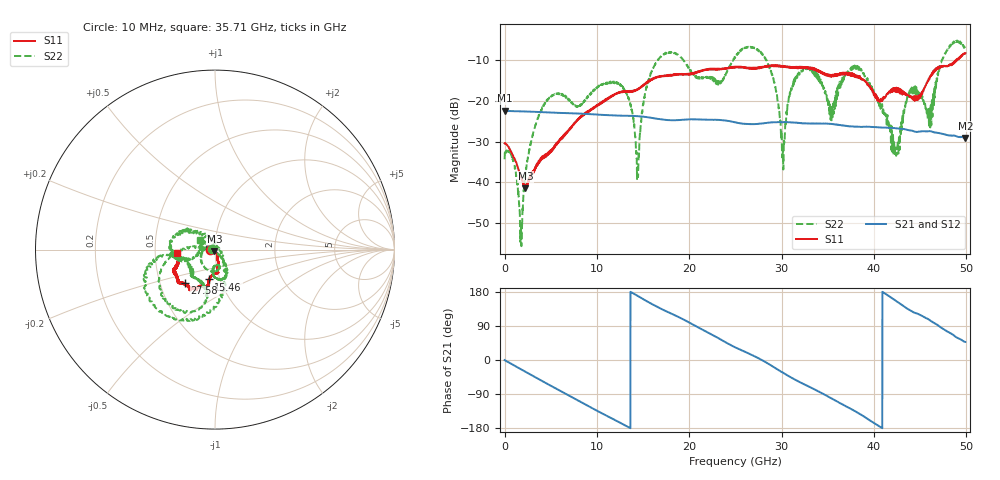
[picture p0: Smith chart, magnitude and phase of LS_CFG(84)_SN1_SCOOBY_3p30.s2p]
!Keysight Technologies,N5245B,MY58422026,A.13.80.08
!Date: Thursday, March 19, 2020 23:53:24
!Correction: S11(Full 2 Port(1,2))
!S21(Full 2 Port(1,2))
!S12(Full 2 Port(1,2))
!S22(Full 2 Port(1,2))
!S2P File: Measurements: S11, S21, S12, S22:
# Hz S DB R 50.0
!freq dBS11 angS11 dBS21 angS21 dBS12 angS12 dBS22 angS22
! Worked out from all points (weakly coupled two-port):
!   4991 points, 10 MHz to 49.91 GHz, reference 50 ohm
!   highest |S21| = -22.43 dB at 10 MHz (marker M1); lowest = -29.1 dB at 49.91 GHz (marker M2)
!   lowest |S11| = -41.5 dB at 2.26 GHz (marker M3), VSWR 1.02, Z = 49.6 - j0.753 ohm
!   |S11| at or under -10 dB: start of sweep to 48.89 GHz; 48.94425 GHz to 48.98609 GHz (41.85 MHz wide, 0.0855 % of centre)
!   |S22| runs from -55.8 to -5.1 dB; largest |S21 - S12| = 0.00076
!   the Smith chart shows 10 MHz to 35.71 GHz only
!   S11 on the Smith chart (normalised r, x): 10 MHz: 0.94, -0.01; 15.46 GHz: 0.88, -0.30; 27.58 GHz: 0.67, -0.27; 35.71 GHz: 0.65, -0.02
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1e7  -30.43 -174.8  -22.43 -0.3  -22.42 -0.3  -34.36 177.2
1.77e9  -38.60 -151.5  -22.54 -24.3  -22.53 -24.2  -52.70 -16.0
2.26e9  -41.47 -115.9  -22.58 -31.0  -22.57 -30.9  -38.36 97.0
4.55e9  -33.19 -61.2  -22.79 -61.8  -22.79 -61.8  -19.82 -140.6
8.33e9  -23.95 -75.8  -23.13 -112.0  -23.13 -111.9  -20.80 -90.5
1.261e10  -17.71 -82.4  -23.63 -166.6  -23.62 -166.6  -16.17 -65.5
1.44e10  -17.02 -94.6  -23.74 169.4  -23.73 169.5  -36.46 -116.3
1.546e10  -15.39 -101.7  -24.01 154.4  -24.00 154.5  -15.48 176.7
1.665e10  -14.10 -100.6  -24.44 138.8  -24.43 138.9  -9.80 -157.9
2.496e10  -11.71 -122.5  -25.23 33.7  -25.22 33.9  -9.26 -168.6
2.758e10  -11.96 -131.8  -25.62 3.7  -25.61 3.9  -7.76 -109.0
3.015e10  -11.46 -142.1  -25.23 -33.5  -25.24 -33.2  -32.97 36.7
3.125e10  -11.62 -147.1  -25.31 -48.9  -25.31 -48.6  -15.48 137.5
3.328e10  -11.96 -155.6  -25.55 -74.3  -25.55 -73.8  -12.27 -173.4
3.571e10  -13.46 -175.5  -25.78 -105.5  -25.71 -105.0  -19.88 147.8
3.817e10  -14.25 173.1  -26.35 -138.1  -26.30 -138.3  -11.39 -173.0
4.16e10  -17.77 107.8  -26.60 169.3  -26.62 169.2  -25.35 74.3
4.245e10  -16.94 105.2  -26.74 155.4  -26.75 155.4  -33.11 -177.9
4.391e10  -18.88 78.6  -27.23 131.5  -27.24 131.7  -17.95 -31.3
4.601e10  -14.62 11.1  -27.41 105.7  -27.43 106.0  -22.81 114.4
4.772e10  -11.41 7.8  -28.26 78.3  -28.28 78.6  -8.23 -79.2
4.991e10  -8.22 -13.4  -29.13 47.5  -29.15 47.7  -7.29 -14.6
